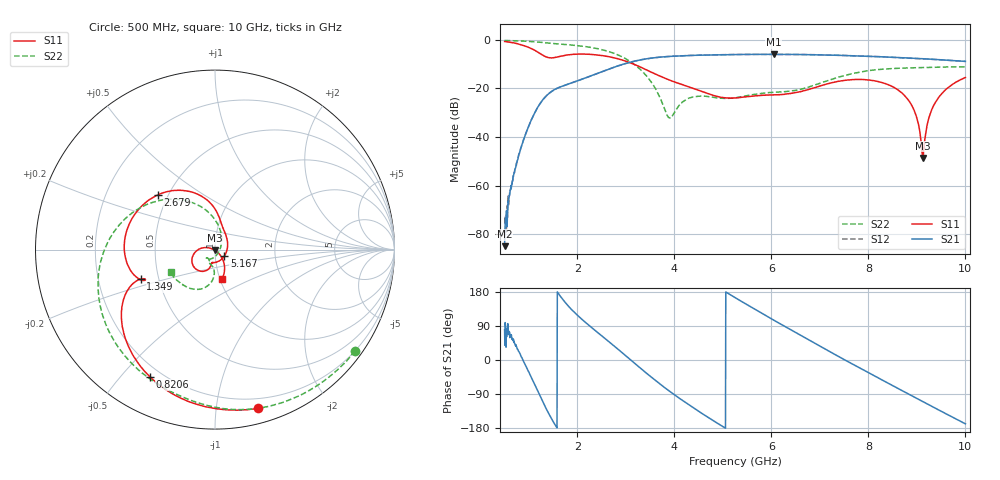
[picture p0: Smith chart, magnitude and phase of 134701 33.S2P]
!  2-Port S-parameters saved by WinCal
! VAR MeasName=S-Parameters (CALIBRATED_DATA) read from VNA (N5242A)
! VAR MeasDate=2013-7-3 16:36:10
! VAR NAME=134701 33
! VAR FILENAME=134701 33.S2P
! VAR DATE=2013-7-3 16:36:10
! VAR PHYS_PORTS=1,2
# Hz S MA R 50
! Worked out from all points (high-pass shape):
!   1601 points, 500 MHz to 10 GHz, reference 50 ohm
!   highest |S21| = -6.04 dB at 6.046 GHz (marker M1); lowest = -84.9 dB at 500 MHz (marker M2)
!   |S21| within 3 dB of the highest: 3.135 GHz to end of sweep
!   lowest |S11| = -48.7 dB at 9.121 GHz (marker M3), VSWR 1.01, Z = 49.8 - j0.298 ohm
!   |S11| at or under -10 dB: 3.152 GHz to end of sweep
!   |S22| runs from -32.2 to -0.3 dB; largest |S21 - S12| = 0.0019
!   S11 on the Smith chart (normalised r, x): 500 MHz: 0.12, -1.30; 820.6 MHz: 0.16, -0.60; 1.349 GHz: 0.40, -0.16; 2.679 GHz: 0.44, +0.33; 5.167 GHz: 1.11, -0.08; 10 GHz: 1.02, -0.34
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5e8  0.9169 -74.8  5.713e-05 80.1  0.0001652 103.5  0.9628 -35.9
6.425e8  0.8746 -94.2  0.001008 64.7  0.0009744 53.8  0.9547 -46.0
8.20625e8  0.7964 -117.0  0.005305 16.2  0.005245 14.8  0.9411 -58.6
1.081875e9  0.6343 -145.4  0.02617 -54.2  0.02613 -54.5  0.9114 -77.2
1.349062e9  0.4448 -158.4  0.06844 -126.4  0.06829 -126.6  0.8609 -95.6
2.085312e9  0.5063 175.6  0.153 108.3  0.1523 108.2  0.7382 -145.2
2.679062e9  0.4405 136.1  0.255 45.3  0.2541 45.4  0.5565 166.9
3.260938e9  0.2848 100.0  0.3773 -17.3  0.3767 -17.2  0.2647 110.7
3.670625e9  0.1844 83.0  0.434 -60.1  0.4335 -60.0  0.0756 61.0
3.908125e9  0.1466 75.5  0.4527 -83.1  0.4526 -83.1  0.02445 -30.1
4.341562e9  0.1036 55.2  0.4737 -122.0  0.4739 -121.9  0.06478 -122.6
5.166875e9  0.06303 -34.1  0.4937 171.2  0.4937 171.2  0.06273 -125.4
5.25e9  0.06354 -44.2  0.4946 164.8  0.4949 164.8  0.0639 -122.4
6.045625e9  0.07335 -100.1  0.499 105.4  0.4983 105.4  0.08264 -110.9
6.835312e9  0.09907 -105.4  0.4916 48.3  0.4921 48.3  0.1121 -93.1
7.565625e9  0.1482 -127.6  0.4702 -3.4  0.4707 -3.5  0.1893 -98.0
8.420625e9  0.1174 -169.9  0.4381 -62.2  0.4367 -62.3  0.2522 -119.8
8.889688e9  0.04554 166.1  0.4167 -93.9  0.4159 -94.0  0.2636 -129.9
9.12125e9  0.003691 -125.8  0.4059 -109.7  0.4049 -109.6  0.2672 -134.2
9.251875e9  0.02567 -46.4  0.3988 -118.5  0.3983 -118.4  0.2687 -136.8
9.394375e9  0.05415 -49.1  0.3916 -128.0  0.3912 -128.0  0.271 -139.5
1e10  0.1669 -76.3  0.3578 -168.4  0.3579 -168.3  0.2761 -152.8
